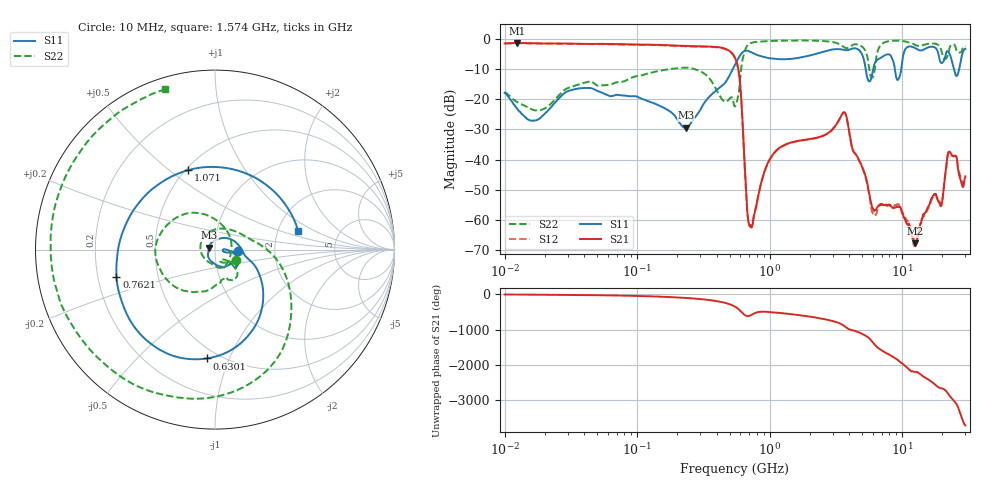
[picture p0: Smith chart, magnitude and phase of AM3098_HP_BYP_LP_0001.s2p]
!Agilent Technologies,E8364B,MY43040894,A.07.50.67
!Agilent E8364B: A.07.50.67
!Date: Wednesday, June 17, 2020 09:19:16
!Correction: S11(Full 2 Port(1,2))
!S21(Full 2 Port(1,2))
!S12(Full 2 Port(1,2))
!S22(Full 2 Port(1,2))
!S2P File: Measurements: S11, S21, S12, S22:Log Frequency Sweep
# Hz S  dB  R 50
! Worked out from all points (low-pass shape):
!   1601 points, 10 MHz to 30 GHz, reference 50 ohm
!   highest |S21| = -1.39 dB at 12.34 MHz (marker M1); lowest = -67.6 dB at 12.5 GHz (marker M2)
!   |S21| within 3 dB of the highest: start of sweep to 509.5 MHz
!   lowest |S11| = -29.4 dB at 233.9 MHz (marker M3), VSWR 1.07, Z = 46.9 + j1.02 ohm
!   |S11| at or under -10 dB: 5.304 GHz to 6.038 GHz (734.1 MHz wide, 12.9 % of centre); 8.814 GHz to 9.846 GHz (1.032 GHz wide, 11.1 % of centre); 24.6 GHz to 26.95 GHz (2.348 GHz wide, 9.11 % of centre)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
!   |S22| runs from -23.7 to -0.6 dB; largest |S21 - S12| = 0.019
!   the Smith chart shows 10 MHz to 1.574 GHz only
!   S11 on the Smith chart (normalised r, x): 10 MHz: 1.29, -0.02; 630.1 MHz: 0.43, -0.83; 762.1 MHz: 0.28, -0.12; 1.071 GHz: 0.51, +0.58; 1.574 GHz: 2.59, +0.69
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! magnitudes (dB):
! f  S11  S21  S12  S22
! 10 MHz  -17.9  -1.6  -1.5  -17.7
! 12.34 MHz  -22.9  -1.4  -1.5  -20.8
! 38.04 MHz  -16.3  -1.7  -1.7  -14.8
! 144.7 MHz  -22.0  -2.0  -2.1  -10.6
! 233.9 MHz  -29.4  -2.4  -2.5  -9.5
! 547.7 MHz  -8.6  -6.3  -6.4  -22.3
! 590.4 MHz  -5.9  -12.3  -12.4  -16.3
! 630.1 MHz  -4.3  -30.8  -31.3  -6.2
! 689.5 MHz  -4.0  -60.2  -59.8  -1.9
! 762.1 MHz  -4.9  -58.4  -58.3  -1.1
! 1.071 GHz  -6.6  -38.0  -38.1  -0.7
! 1.574 GHz  -6.5  -33.9  -33.9  -0.6
! 2.084 GHz  -5.4  -33.0  -33.1  -0.6
! 3.668 GHz  -3.7  -24.3  -24.4  -2.9
! 6.049 GHz  -9.8  -56.4  -58.1  -12.4
! 7.926 GHz  -5.2  -54.8  -55.0  -0.8
! 9.302 GHz  -13.5  -55.5  -54.6  -0.6
! 12.5 GHz  -3.0  -67.6  -68.5  -2.0
! 19.7 GHz  -8.0  -55.2  -55.1  -3.7
! 22.67 GHz  -4.8  -37.3  -37.6  -3.3
! 25.82 GHz  -12.3  -39.4  -39.6  -4.1
! 30 GHz  -3.3  -45.5  -46.3  -2.5
